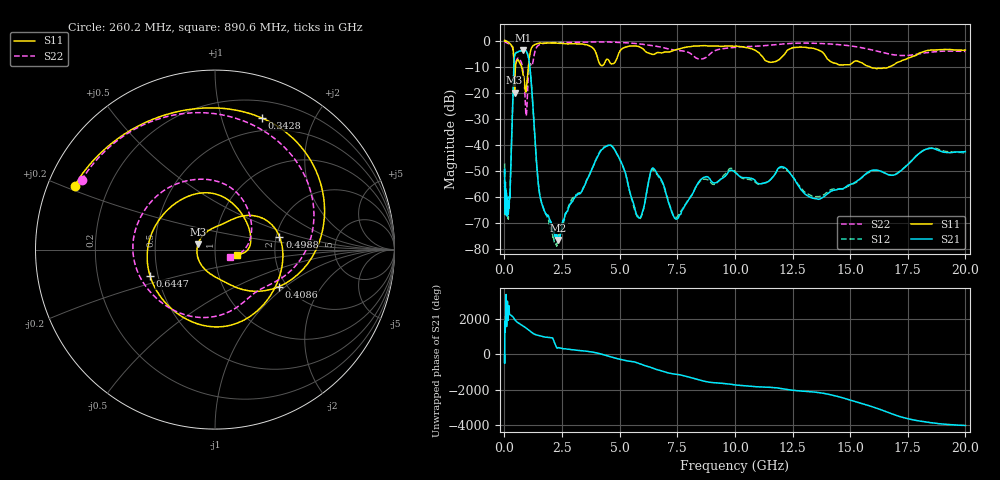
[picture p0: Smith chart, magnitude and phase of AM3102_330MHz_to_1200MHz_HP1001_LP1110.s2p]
! Date/Time: Tue, Sep 11, 2018 5:18 PM
! Network Analyzer: Agilent Technologies E8362B Rev: A.07.50.63
! Sweep from 0.010 to 20.000 GHz, 1601 Points, Sweep Type: LOG
! Power Supply: 4.949 V, 0.001 A
# Hz S DB R 50
!freq MagS11 AngS11 MagS21 AngS21 MagS12 AngS12 MagS22 AngS22
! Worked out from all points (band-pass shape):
!   1601 points, 10 MHz to 20 GHz, reference 50 ohm
!   highest |S21| = -3.59 dB at 817.6 MHz (marker M1); lowest = -76.6 dB at 2.336 GHz (marker M2)
!   |S21| within 3 dB of the highest: 433.4 MHz to 1.046 GHz (613 MHz wide, 82.9 % of centre)
!   lowest |S11| = -20.0 dB at 443 MHz (marker M3), VSWR 1.22, Z = 41.3 + j2.54 ohm
!   |S11| at or under -10 dB: 415.6 MHz to 480.2 MHz (64.65 MHz wide, 14.4 % of centre); 745.5 MHz to 1.041 GHz (295.7 MHz wide, 33.1 % of centre); 15.84 GHz to 16.72 GHz (886.1 MHz wide, 5.44 % of centre)
!   |S22| runs from -28.9 to -0.2 dB; largest |S21 - S12| = 0.0091
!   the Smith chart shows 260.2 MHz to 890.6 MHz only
!   S11 on the Smith chart (normalised r, x): 260.2 MHz: 0.08, +0.21; 342.8 MHz: 0.36, +1.35; 408.6 MHz: 1.82, -0.90; 498.8 MHz: 2.08, +0.35; 644.7 MHz: 0.45, -0.16; 890.6 MHz: 1.28, -0.08
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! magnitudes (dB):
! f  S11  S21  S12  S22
! 10 MHz  0.0  -51.1  -47.2  -0.2
! 35.55 MHz  0.0  -61.7  -64.8  -0.5
! 126.4 MHz  -0.4  -62.2  -62.1  -1.0
! 260.2 MHz  -1.3  -53.8  -54.4  -1.5
! 342.8 MHz  -2.2  -29.4  -29.5  -2.5
! 408.6 MHz  -7.7  -10.4  -10.4  -6.1
! 443 MHz  -20.0  -5.8  -5.9  -9.6
! 447.2 MHz  -19.8  -5.6  -5.7  -9.7
! 498.8 MHz  -8.7  -4.8  -4.8  -8.2
! 644.7 MHz  -8.2  -4.1  -4.2  -7.1
! 817.6 MHz  -13.3  -3.6  -3.7  -12.2
! 890.6 MHz  -17.8  -3.6  -3.7  -20.4
! 1.124 GHz  -4.4  -11.8  -11.8  -8.9
! 1.59 GHz  -1.0  -61.5  -61.4  -1.3
! 2.336 GHz  -1.0  -76.6  -76.4  -0.8
! 4.436 GHz  -7.2  -40.6  -40.5  -0.5
! 5.652 GHz  -2.1  -64.1  -65.1  -1.1
! 6.518 GHz  -5.2  -49.5  -50.1  -2.1
! 7.517 GHz  -3.4  -68.3  -67.6  -3.8
! 8.627 GHz  -1.9  -52.7  -53.3  -7.0
! 13.61 GHz  -3.6  -61.0  -59.9  -1.1
! 20 GHz  -3.7  -42.7  -43.2  -4.2
